(* Logix 5000 AddOnInstructionDefinition export MIS_COM; software revision 33.00 *)

TYPE JVL_AXIS_MIS :   // Drive Data
STRUCT
   ActualMode : DINT;
   ActualPosition : REAL;   // P_IST
   ActualVelocity : REAL;   // V_IST(16)
   ActualTorque : REAL;   // ACTUAL_TORQUE
   AxisStatus : JVL_MIS_STATUS;
   AxisWarnings : JVL_MIS_Warnings;
   AxisError : JVL_MIS_Error;
   RequestedMode : DINT;
   RequestedPosition : DINT;   // P_SOLL
   RequestedVelocity : DINT;   // V_SOLL
   RequestedAcceleration : DINT;   // A_SOLL
   RequestedDeceleration : DINT;
   GeneralCommand : DINT;
   CommandTorque : REAL;   // Requested Torque, T_SOLL
   ZeroSearchVelocity : REAL;   // Homing velocity
   ZeroSearchPosition : REAL;   // Homing position
   ZeroSearchTorque : DINT;   // Homing torque setpoint threshold value
   ZeroSearchTThreshold : DINT;   // Threshold for torque zerosearch trigger, usually 20% lower than running torque
   TravelConst : REAL;   // Factor to multiply P_IST and P_SOLL for scaling
   VelConst : REAL;   // Factor to multiply V_SOLL and V_IST to get scaled velocity value
   HomingType : DINT;   // Holds the reqested homingtype
   LoadFactor : DINT;   // Inertia ratio motor/load
   Configured : DINT;
   MSG_OutValue : DINT;   // Used in exp. output message to the motor
   MSG_InValue : DINT;   // Used in Exp. output message, to get value from motor
   MSG_OutInstance : DINT;   // Registernumber
   MSG_InInstance : DINT;   // Registernummer
   V_SOLL_CountsPerSample : REAL;
   AOI_Type : DINT;   // MIS_Disable = 1, MIS_Home = 2, MIS_Jog = 3, MIS_Position = 4, MIS_Reset = 5, MIS_Stop = 6
   Position_AppType : REAL;   // Position depending on the Application type
   MSG_Out_Execute : BOOL;   // Enable MSG_Out
   MSG_In_Execute : BOOL;   // Enable MSG_In
   ErrorReset : BOOL;
   MSG_Out_Busy : BOOL;
   MSG_In_Busy : BOOL;
   MSG_Out_Done : BOOL;
   MSG_In_Done : BOOL;
END_STRUCT
END_TYPE

TYPE JVL_MIS_Error :
STRUCT
   GeneralError : BOOL;
   FollowingError : BOOL;
   OutputDriver : BOOL;
   PositionLimit : BOOL;
   LowBusVoltage : BOOL;
   OverVoltage : BOOL;
   TemperatureLimit : BOOL;
   Internal : BOOL;
   AbsoluteMultiturnEncoderPositionLost : BOOL;
   AbsoluteMultiturnEncoderSensorCounting : BOOL;
   AbsoluteMultiturnEncoderCommsFailed : BOOL;
   SSIEncoderCounting : BOOL;
   ClosedLoop : BOOL;
   ExternalMemory : BOOL;
   AbsoluteSingleturnEncoder : BOOL;
   H4InternalEncoderError : BOOL;
   ZeroSearchTimeout : BOOL;
   CVIUnstable : BOOL;
   MotorDriverOverload : BOOL;
   Reserved_19 : BOOL;
   Reserved_20 : BOOL;
   Reserved_21 : BOOL;
   Reserved_22 : BOOL;
   Reserved_23 : BOOL;
   Reserved_24 : BOOL;
   Reserved_25 : BOOL;
   Reserved_26 : BOOL;
   STO_Alarm : BOOL;
   Reserved_28 : BOOL;
   STO : BOOL;
   Reserved_30 : BOOL;
   Reserved_31 : BOOL;
END_STRUCT
END_TYPE

TYPE JVL_MIS_STATUS :   // STATUS JVL Stepper
STRUCT
   Reserved_0 : BOOL;
   AutoCorrectionActive : BOOL;
   InPhysicalPosition : BOOL;
   AtVelocity : BOOL;
   InPosition : BOOL;
   Accelerating : BOOL;
   Decelerating : BOOL;
   ZeroSearchDone : BOOL;
   PasswordLock : BOOL;
   MagneticEncoderError : BOOL;
   H3CalibrationDataPresent : BOOL;
   H3LinearisationTableRecorded : BOOL;
   GeneralError : BOOL;
   H3CalibrationDataLocked : BOOL;
   ElectromechBrakeActive : BOOL;
   ClosedLoopLeadLagDetected : BOOL;
   ClosedLoopActivated : BOOL;
   InternalEncoderCalibrated : BOOL;
   StandbyCurrentIsUsed : BOOL;
   STOEnabled : BOOL;
   InternalEncoderOK : BOOL;
   EthernetSyncActivated : BOOL;
   InTargetPosition : BOOL;
   STOChannelAOK : BOOL;
   STOChannelBOK : BOOL;
   External_memory_sizeA : BOOL;
   External_memory_sizeB : BOOL;
   Reserved_27 : BOOL;
   Reserved_28 : BOOL;
   Reserved_29 : BOOL;
   Reserved_30 : BOOL;
   Reserved_31 : BOOL;
END_STRUCT
END_TYPE

TYPE JVL_MIS_Warnings :
STRUCT
   PositiveLimitActive : BOOL;
   NegativeLimitActive : BOOL;
   PositiveLimitHasBeenReached : BOOL;
   NegativeLimitHasBeenReached : BOOL;
   LowBusVoltage : BOOL;
   Reserved_5 : BOOL;
   TemperatureWarning : BOOL;
   SSIEncoder : BOOL;
   DriverOverload : BOOL;
   STOActive : BOOL;
   Reserved_10 : BOOL;
   Reserved_11 : BOOL;
   Reserved_12 : BOOL;
   Reserved_13 : BOOL;
   Reserved_14 : BOOL;
   Reserved_15 : BOOL;
   Reserved_16 : BOOL;
   Reserved_17 : BOOL;
   Reserved_18 : BOOL;
   Reserved_19 : BOOL;
   Reserved_20 : BOOL;
   Reserved_21 : BOOL;
   Reserved_22 : BOOL;
   Reserved_23 : BOOL;
   Reserved_24 : BOOL;
   Reserved_25 : BOOL;
   Reserved_26 : BOOL;
   Reserved_27 : BOOL;
   Reserved_28 : BOOL;
   Reserved_29 : BOOL;
   Reserved_30 : BOOL;
   Reserved_31 : BOOL;
END_STRUCT
END_TYPE

ADD_ON_INSTRUCTION MIS_COM   (* revision 1.0 *)
VAR_IN_OUT
   JVL_IN : AB:ETHERNET_MODULE_DINT_32Bytes:I:0; {required}
   JVL_OUT : AB:ETHERNET_MODULE_DINT_32Bytes:O:0; {required}
   MSG_IN : MESSAGE; {required}
   MSG_OUT : MESSAGE; {required}
   AXIS : JVL_AXIS_MIS; {required}
END_VAR
VAR_INPUT
   TravelPerRev : REAL := 1.0; {required}   // Travel per Revolution. Exc. actuator w. 60mm/rev, then value=60
   GearRatio : REAL := 1.0; {required}   // Gear ratio if a gearbox is mounted. select 1 for none
   ApplicationType : DINT; {required}   // Application_Type - 0=none (counts) 1=linear 2=degree
END_VAR
VAR
   CountsPerRevolution : REAL; {access None}
   vel : INT; {access None}
   torque : INT; {access None}
END_VAR

ROUTINE Logic   (* structured text *)
   
   
   	    AXIS.V_SOLL_CountsPerSample := 100.0;
   		CountsPerRevolution:= 409600.0;
   
   
   	//counts
   	if ApplicationType = 0 then
   	AXIS.TravelConst := 1;
   	AXIS.VelConst:= AXIS.V_SOLL_CountsPerSample;
   	//linear
   	elsif ApplicationType = 1 then
   	AXIS.TravelConst :=(CountsPerRevolution * GearRatio) / TravelPerRev;
   	AXIS.VelConst:= AXIS.V_SOLL_CountsPerSample * 60 * GearRatio / TravelPerRev;
   	//360°
   	elsif ApplicationType = 2 then
   	AXIS.TravelConst :=(CountsPerRevolution * GearRatio) / 360;
   	AXIS.VelConst:= AXIS.V_SOLL_CountsPerSample * 60 * GearRatio / 360;
   	end_if;
   
   
   AXIS.ActualMode := JVL_IN.Data[0];
   AXIS.ActualPosition := JVL_IN.Data[1];
   AXIS.ActualVelocity := JVL_IN.Data[2]/AXIS.VelConst;
   
   AXIS.ActualTorque := abs(JVL_IN.Data[6]) *0.049; //* 100 / 2047;
   
   AXIS.Position_AppType := AXIS.ActualPosition /AXIS.TravelConst;
   JVL_OUT.Data[0]:= AXIS.RequestedMode;
   //cop(AXIS.RequestedPosition,JVL_OUT.Data[1],4);
   JVL_OUT.Data[1]:= AXIS.RequestedPosition;
   //cop(AXIS.RequestedVelocity,JVL_OUT.Data[2],4);
   JVL_OUT.Data[2]:= AXIS.RequestedVelocity;
   JVL_OUT.Data[3]:= AXIS.RequestedAcceleration;
   JVL_OUT.Data[4]:= AXIS.RequestedDeceleration;
   JVL_OUT.Data[5]:= AXIS.GeneralCommand;
   
   AXIS.MSG_Out_Done:= MSG_OUT.DN;
   AXIS.MSG_Out_Busy:= MSG_OUT.EN;
   AXIS.MSG_In_Done:= MSG_IN.DN;
   AXIS.MSG_In_Busy:= MSG_IN.EN;
   
   MSG_OUT.Instance:= AXIS.MSG_OutInstance;
   MSG_IN.Instance:= AXIS.MSG_InInstance;
   //Status
     AXIS.AxisStatus.STOChannelBOK := JVL_IN.Data[3].24;
     AXIS.AxisStatus.External_memory_sizeA := JVL_IN.Data[3].25;
     AXIS.AxisStatus.External_memory_sizeB := JVL_IN.Data[3].26;
     AXIS.AxisStatus.Reserved_27 := JVL_IN.Data[3].27;
     AXIS.AxisStatus.Reserved_28 := JVL_IN.Data[3].28;
     AXIS.AxisStatus.Reserved_29 := JVL_IN.Data[3].29;
     AXIS.AxisStatus.Reserved_30 := JVL_IN.Data[3].30;
     AXIS.AxisStatus.Reserved_31 := JVL_IN.Data[3].31;
     AXIS.AxisStatus.ClosedLoopActivated := JVL_IN.Data[3].16;
     AXIS.AxisStatus.InternalEncoderCalibrated := JVL_IN.Data[3].17;
     AXIS.AxisStatus.StandbyCurrentIsUsed := JVL_IN.Data[3].18;
     AXIS.AxisStatus.STOEnabled := JVL_IN.Data[3].19;
     AXIS.AxisStatus.InternalEncoderOK := JVL_IN.Data[3].20;
     AXIS.AxisStatus.EthernetSyncActivated := JVL_IN.Data[3].21;
     AXIS.AxisStatus.InTargetPosition := JVL_IN.Data[3].22;
     AXIS.AxisStatus.STOChannelAOK := JVL_IN.Data[3].23;
     AXIS.AxisStatus.PasswordLock := JVL_IN.Data[3].8;
     AXIS.AxisStatus.MagneticEncoderError := JVL_IN.Data[3].9;
     AXIS.AxisStatus.H3CalibrationDataPresent := JVL_IN.Data[3].10;
     AXIS.AxisStatus.H3LinearisationTableRecorded := JVL_IN.Data[3].11;
     AXIS.AxisStatus.GeneralError := JVL_IN.Data[3].12;
     AXIS.AxisStatus.H3CalibrationDataLocked := JVL_IN.Data[3].13;
     AXIS.AxisStatus.ElectromechBrakeActive := JVL_IN.Data[3].14;
     AXIS.AxisStatus.ClosedLoopLeadLagDetected := JVL_IN.Data[3].15;
     AXIS.AxisStatus.Reserved_0 := JVL_IN.Data[3].0;
     AXIS.AxisStatus.AutoCorrectionActive := JVL_IN.Data[3].1;
     AXIS.AxisStatus.InPhysicalPosition := JVL_IN.Data[3].2;
     AXIS.AxisStatus.AtVelocity := JVL_IN.Data[3].3;
     AXIS.AxisStatus.InPosition := JVL_IN.Data[3].4;
     AXIS.AxisStatus.Accelerating := JVL_IN.Data[3].5;
     AXIS.AxisStatus.Decelerating := JVL_IN.Data[3].6;
     AXIS.AxisStatus.ZeroSearchDone := JVL_IN.Data[3].7;
   
     //Warnings
   AXIS.AxisWarnings.PositiveLimitActive := JVL_IN.Data[4].0;
   AXIS.AxisWarnings.NegativeLimitActive := JVL_IN.Data[4].1;
   AXIS.AxisWarnings.PositiveLimitHasBeenReached := JVL_IN.Data[4].2;
   AXIS.AxisWarnings.NegativeLimitHasBeenReached := JVL_IN.Data[4].3;
   AXIS.AxisWarnings.LowBusVoltage := JVL_IN.Data[4].4;
   AXIS.AxisWarnings.Reserved_5 := JVL_IN.Data[4].5;
   AXIS.AxisWarnings.TemperatureWarning := JVL_IN.Data[4].6;
   AXIS.AxisWarnings.SSIEncoder := JVL_IN.Data[4].7;
   AXIS.AxisWarnings.DriverOverload := JVL_IN.Data[4].8;
   AXIS.AxisWarnings.STOActive := JVL_IN.Data[4].9;
   
   //ErrorsAXIS.AxisError.Reserved_24 := JVL_IN.Data[5].24;
   AXIS.AxisError.Reserved_25 := JVL_IN.Data[5].25;
   AXIS.AxisError.Reserved_26 := JVL_IN.Data[5].26;
   AXIS.AxisError.STO_Alarm := JVL_IN.Data[5].27;
   AXIS.AxisError.Reserved_28 := JVL_IN.Data[5].28;
   AXIS.AxisError.STO := JVL_IN.Data[5].29;
   AXIS.AxisError.Reserved_30 := JVL_IN.Data[5].30;
   AXIS.AxisError.Reserved_31 := JVL_IN.Data[5].31;
   AXIS.AxisError.ZeroSearchTimeout := JVL_IN.Data[5].16;
   AXIS.AxisError.CVIUnstable := JVL_IN.Data[5].17;
   AXIS.AxisError.MotorDriverOverload := JVL_IN.Data[5].18;
   AXIS.AxisError.Reserved_19 := JVL_IN.Data[5].19;
   AXIS.AxisError.Reserved_20 := JVL_IN.Data[5].20;
   AXIS.AxisError.Reserved_21 := JVL_IN.Data[5].21;
   AXIS.AxisError.Reserved_22 := JVL_IN.Data[5].22;
   AXIS.AxisError.Reserved_23 := JVL_IN.Data[5].23;
   AXIS.AxisError.AbsoluteMultiturnEncoderPositionLost := JVL_IN.Data[5].8;
   AXIS.AxisError.AbsoluteMultiturnEncoderSensorCounting := JVL_IN.Data[5].9;
   AXIS.AxisError.AbsoluteMultiturnEncoderCommsFailed := JVL_IN.Data[5].10;
   AXIS.AxisError.SSIEncoderCounting := JVL_IN.Data[5].11;
   AXIS.AxisError.ClosedLoop := JVL_IN.Data[5].12;
   AXIS.AxisError.ExternalMemory := JVL_IN.Data[5].13;
   AXIS.AxisError.AbsoluteSingleturnEncoder := JVL_IN.Data[5].14;
   AXIS.AxisError.H4InternalEncoderError := JVL_IN.Data[5].15;
   AXIS.AxisError.GeneralError := JVL_IN.Data[5].0;
   AXIS.AxisError.FollowingError := JVL_IN.Data[5].1;
   AXIS.AxisError.OutputDriver := JVL_IN.Data[5].2;
   AXIS.AxisError.PositionLimit := JVL_IN.Data[5].3;
   AXIS.AxisError.LowBusVoltage := JVL_IN.Data[5].4;
   AXIS.AxisError.OverVoltage := JVL_IN.Data[5].5;
   AXIS.AxisError.TemperatureLimit := JVL_IN.Data[5].6;
   AXIS.AxisError.Internal := JVL_IN.Data[5].7;
   
END_ROUTINE
END_ADD_ON_INSTRUCTION

ADD_ON_INSTRUCTION MIS_Disable   (* revision 1.0 *)
VAR_IN_OUT
   AXIS : JVL_AXIS_MIS; {required}
END_VAR
VAR_OUTPUT
   Busy : BOOL; {access Read Only, visible}
   CommandAborted : BOOL; {access Read Only, visible}
   Done : BOOL; {access Read Only, visible}
   Error : BOOL; {access Read Only, visible}
END_VAR
VAR_INPUT
   Execute : BOOL; {required}
END_VAR
VAR
   State : INT; {access None}
   ExecuteStart : BOOL; {access None}
   AOI_Type : DINT; {access None}
END_VAR

ROUTINE Logic   (* structured text *)
   	//REGION CAPTURE EDGES
   	    if Execute and not ExecuteStart then
   	    	ExecuteStart:=1;
   		elsif not Execute then
   			ExecuteStart:=0;
   		end_if;
   
   	//END_REGION
   
   	//REGION STATE CHANGES
   
   	    //Re-trigger sequence from start on rising edge
   
   	    //Command aborted
   	    IF AXIS.AOI_Type <> AOI_Type AND
   	        State <> 0 AND
   	        State <> 90 AND
   	        State <> 30 AND
   	        State <> 80
   	    THEN
   	        State := 80;
   	    END_IF;
   
   
   	    //Error if motor error while executing
   	    IF AXIS.AxisError.GeneralError AND
   	        State <> 0 AND
   	        State <> 90 AND
   	        State <> 20 AND
   	        State <> 80
   	    THEN
   	        State := 90;
   	    END_IF;
   
   	//END_REGION
   
   	//REGION STATE MACHINE
   
   	    CASE State OF
   
   	        0:        //Wait for rising edge on execute
   	            IF ExecuteStart THEN
   					AOI_Type:= 1;
   					AXIS.AOI_Type:= 1;
   	                State := 10;
   	            END_IF;
   
   	        10:     //Put JVL into passive state
   	            AXIS.RequestedMode:= 0;
   	            IF AXIS.ActualMode = 0 THEN
   	                State := 20;
   	            END_IF;
   
   	        20:        //Disable complete, reset to idle by setting execute false
   	            IF NOT Execute THEN
   	                State := 0;
   	            END_IF;
   
   	        80:     //Aborted by other command before completion
   	            IF NOT Execute THEN
   	                State := 0;
   	            END_IF;
   
   	        90:       //Error while disabling, reset to idle by setting execute false
   	            IF NOT Execute THEN
   	                State := 0;
   	            END_IF;
   
   	        ELSE
   	            State := 90;
   
   	    END_CASE;
   
   	//END_REGION
   
   	//REGION STATUS SIGNALS
   
   	    Done := State = 20;
   	    CommandAborted := State = 80;
   	    Error := State = 90;
   	    Busy := State <> 0 AND NOT Done AND NOT Error AND NOT CommandAborted;
   
   	//END_REGION
   
END_ROUTINE
END_ADD_ON_INSTRUCTION

ADD_ON_INSTRUCTION MIS_Home   (* revision 1.0 *)
VAR_IN_OUT
   Axis : JVL_AXIS_MIS; {required}
END_VAR
VAR_OUTPUT
   Busy : BOOL; {access Read Only, visible}
   CommandAborted : BOOL; {access Read Only, visible}
   Done : BOOL; {access Read Only, visible}
   Error : BOOL; {access Read Only, visible}
END_VAR
VAR_INPUT
   Execute : BOOL; {required}
   Mode : INT; {required}
   Position : REAL; {required}
   Offset : REAL; {required}
   Velocity : REAL; {required}
   VelocityReduced : REAL; {required}
   Acceleration : REAL; {required}
   Deceleration : REAL; {required}
   TorqueLimit : REAL; {required}
END_VAR
VAR
   State : INT; {access None}
   ActiveMode : INT; {access None}
   Mode0State : INT; {access None}
   Mode1State : INT; {access None}
   ActivePosition : REAL; {access None}
   ActiveVelocity : REAL; {access None}
   ActiveAcceleration : REAL; {access None}
   ActiveTorqueLimit : REAL; {access None}
   ActiveOffset : REAL; {access None}
   Mode2State : INT; {access None}
   Mode3State : INT; {access None}
   ExecuteStart : BOOL; {access None}
   Ton_wait : FBD_TIMER; {access None}
   AOI_Type : DINT; {access None}
   ActiveVelocityReduced : REAL;
   ActiveDeceleration : DINT; {access None}
END_VAR

ROUTINE Logic   (* structured text *)
   	//REGION CAPTURE EDGES
   	    if Execute and not ExecuteStart then
   	    	ExecuteStart:=1;
   		elsif not Execute then
   			ExecuteStart:=0;
   		end_if;
   
   	//END_REGION
   
   	//REGION STATE CHANGES
   
   	    //Re-trigger sequence from start on rising edge
   
   
   	    //Command aborted
   	    IF Axis.AOI_Type <> AOI_Type AND
   	        State <> 0 AND
   	        State <> 90 AND
   	        State <> 30 AND
   	        State <> 80
   	    THEN
   	        State := 80;
   	    END_IF;
   
   
   	    //Error if motor error while executing
   	    IF Axis.AxisError.GeneralError AND
   	        State <> 0 AND
   	        State <> 90 AND
   	        State <> 30 AND
   	        State <> 80
   	    THEN
   	        State := 90;
   	    END_IF;
   	//END_REGION
   
   	//REGION STATE MACHINE
   
   
   
   	    CASE State OF
   
   	        0:
   	            //Reset static values
   	            ActiveMode := 0;
   	            ActivePosition := 0;
   	            ActiveVelocity := 0;
   	            ActiveVelocityReduced:=0;
   				ActiveAcceleration := 0;
   	            ActiveDeceleration := 0;
   				ActiveTorqueLimit := 0;
   	            ActiveOffset := 0;
   
   	            //Reset mode states
   	            Mode0State := 0;
   	            Mode1State := 0;
   	            Mode2State := 0;
   	            Mode3State := 0;
   
   	            IF ExecuteStart THEN
   					//
   					AOI_Type:= 2;
   					Axis.AOI_Type:= 2;
   	                //
   					Axis.GeneralCommand := 0;
   	                ActiveMode := Mode;
   	                ActivePosition := Position * Axis.TravelConst;
   	                ActiveVelocity := Velocity * Axis.VelConst;// * Axis.Device.Config.V_SOLL_CountsPerSample);
   	                ActiveVelocityReduced := VelocityReduced * Axis.VelConst;// * Axis.Device.Config.V_SOLL_CountsPerSample);
   	                ActiveAcceleration := ABS(Acceleration) ;
   	                ActiveDeceleration := ABS(Deceleration) ;
   	                //set Acceleration always >=1
   	                IF ActiveAcceleration < 1 THEN
   	                    ActiveAcceleration := 1;
   	                END_IF;
   
   	                ActiveTorqueLimit := TorqueLimit * 2047/100;
   	                ActiveOffset := Offset * Axis.TravelConst;
   
   	                State := 10;
   	            END_IF;
   
   	        10:
   	            // change to velocity mode with zero setpoint to ensure motor does not run off to current position when homed
   	            IF ActiveAcceleration < 1 THEN
   	                Axis.RequestedAcceleration := 1;
   	            ELSE
   	                Axis.RequestedAcceleration := ActiveAcceleration;
   	                Axis.RequestedDeceleration := ActiveDeceleration;
   
   	            END_IF;
   	            Axis.RequestedVelocity := 0;
   	            Axis.RequestedMode := 1;
   	            // change position setpoint to new home position
   	            Axis.RequestedPosition := ActivePosition;
   	            // reset register trigger
   	            Axis.MSG_Out_Execute := 0;
   	            Axis.MSG_In_Execute := 0;
   	            // start homing
   	            State := 20;
   
   	        20:
   	            CASE ActiveMode OF
   
   	                0:  // Set Home Position
   	                    CASE Mode0State OF
   	                        0:
   
   								Axis.MSG_OutInstance := 144;
   
   	                            Axis.MSG_OutValue:=Position;
   	                            Axis.MSG_Out_Execute := 1;
   	                            Axis.GeneralCommand := 16#0;
   	                            IF Axis.MSG_Out_Busy AND NOT Axis.MSG_Out_Done THEN
   	                                Mode0State := 10;
   	                            END_IF;
   	                        10:
   	                            IF Axis.MSG_Out_Done THEN
   	                                Axis.MSG_Out_Execute := 0;
   	                                Mode0State := 20;
   	                            END_IF;
   	                        20:
   	                            Axis.GeneralCommand := 16#80000162;//16#1000162 also
   	                            IF ABS(Axis.ActualPosition - Position) < 50.0 THEN
   	                                Mode0State := 30;
   	                            END_IF;
   	                        30:
   	                            Axis.GeneralCommand := 16#0;
   	                            Mode0State := 50;
   	                        50:
   	                            State := 30;
   	                        ELSE
   	                            State := 90;
   	                    END_CASE;
   
   	                1:  // Home to Sensor (type 2, bidirectional)
   	                    CASE Mode1State OF
   	                       0:
   	                            // set home position offset move distance
   
   		                            Axis.MSG_OutInstance := 38;
   		                            Axis.MSG_OutValue := ActiveOffset;
   		                            Axis.MSG_Out_Execute := 1;
   		                            IF Axis.MSG_Out_Busy THEN
   		                                Mode1State := 5;
   		                            END_IF;
   
   	                        5:
   
   	                            IF Axis.MSG_Out_Done THEN
   	                                Axis.MSG_Out_Execute := 0;
   	                                Mode1State := 10;
   	                            END_IF;
   	                       10:
   	                            //homing velocity
   	                            Axis.MSG_OutInstance := 40;
   	                            Axis.MSG_OutValue:=ActiveVelocity;
   
   	                            Axis.MSG_Out_Execute := 1;
   	                            IF Axis.MSG_Out_Busy THEN
   	                                Mode1State := 15;
   	                            END_IF;
   	                       15:
   	                            IF Axis.MSG_Out_Done THEN
   	                                Axis.MSG_Out_Execute := 0;
   	                                Mode1State := 20;
   	                            END_IF;
   
   	                       20:
   	                            // set homing reduced/crawl velocity
   	                            Axis.MSG_OutInstance := 242;
   	                            Axis.MSG_OutValue:=ActiveVelocityReduced;
   	                            Axis.MSG_Out_Execute := 1;
   	                            IF Axis.MSG_Out_Busy THEN
   	                                Mode1State := 30;
   	                            END_IF;
   	                        30:
   	                            IF Axis.MSG_Out_Done THEN
   	                                Axis.MSG_Out_Execute := 0;
   	                                Mode1State := 60;
   	                            END_IF;
   	                        60:
   	                            // start homing mode
   	                            Axis.RequestedMode := 14;
   
   	                            // homing done
   	                            IF NOT Axis.AxisStatus.ZeroSearchDone THEN
   	                                Mode1State := 70;
   	                            END_IF;
   	                        70:
   	                            IF Axis.AxisStatus.ZeroSearchDone THEN
   	                                Axis.RequestedVelocity := 0;
   	                                Axis.RequestedMode := 2;
   	                                Mode1State := 80;
   	                            END_IF;
   	                        80:
   	                            State := 30;
   	                        ELSE
   	                            State := 90;
   	                    END_CASE;
   
   	                2:  // Home to Endstop (torque limit)
   	                    CASE Mode2State OF
   	                        0:
   	                            //Home to Endstop (torque limit);
   								Axis.MSG_OutInstance := 38;
   	                            Axis.MSG_OutValue := ActiveOffset;
   	                            Axis.MSG_Out_Execute := 1;
   
   	                            IF Axis.MSG_Out_Busy THEN
   	                                Mode2State := 15;
   	                            END_IF;
   	                        15:
   	                            IF Axis.MSG_Out_Done THEN
   	                                Axis.MSG_Out_Execute := 0;
   	                                Mode2State := 20;
   	                            END_IF;
   	                        20:
   								Axis.MSG_OutInstance := 40;
   	                            Axis.MSG_OutValue := ActiveVelocity;// * Axis.Device.Config.V_SOLL_CountsPerSample;
   	                            Axis.MSG_Out_Execute := 1;
   	                            IF Axis.MSG_Out_Busy THEN
   	                                Mode2State := 25;
   	                            END_IF;
   	                        25:
   	                            IF Axis.MSG_Out_Done THEN
   	                                Axis.MSG_Out_Execute := 0;
   	                                Mode2State := 34;
   
   	                            END_IF;
   	                        34:
   								Axis.MSG_OutInstance := 41;
   	                            Axis.MSG_OutValue := ActiveTorqueLimit;
   	                            Axis.MSG_Out_Execute := 1;
   
   	                            IF Axis.MSG_Out_Busy THEN
   	                                Mode2State := 37;
   	                            END_IF;
   	                        37:
   	                            IF Axis.MSG_Out_Done THEN
   	                                Axis.MSG_Out_Execute := 0;
   	                                Mode2State := 40;
   	                            END_IF;
   	                        40:
   	                            Axis.RequestedMode := 12;
   	                            // homing done-register 42 Homemode bit 16
   	                            IF NOT Axis.AxisStatus.ZeroSearchDone THEN
   	                                Mode2State := 45;
   	                            END_IF;
   	                        45:
   	                            IF Axis.AxisStatus.ZeroSearchDone THEN
   	                                Axis.RequestedVelocity := 0;
   	                                Axis.RequestedMode := 2;
   	                                Mode2State := 60;
   	                            END_IF;
   
   	                        60:
   	                            State := 30;
   	                        ELSE
   	                            State := 90;
   	                    END_CASE;
   
   
   
   	            END_CASE;
   
   	        30:        //Home complete, reset to idle by setting execute false
   	            IF NOT Execute THEN
   	                State := 0;
   	            END_IF;
   
   	        80:     //Aborted by other command before completion
   	            IF NOT Execute THEN
   	                State := 0;
   	            END_IF;
   
   	        90:       //Error while disabling, reset to idle by setting execute false
   	            IF NOT Execute THEN
   	                State := 0;
   	            END_IF;
   
   	        ELSE
   	            State := 90;
   
   	    END_CASE;
   
   	//END_REGION
   
   	//REGION STATUS SIGNALS
   
   	    Done := State = 30;
   	    CommandAborted := State = 80;
   	    Error := State = 90;
   	    Busy := State <> 0 AND NOT Done AND NOT Error AND NOT CommandAborted;
   
   	//END_REGION
END_ROUTINE
END_ADD_ON_INSTRUCTION

ADD_ON_INSTRUCTION MIS_Jog   (* revision 1.0 *)
VAR_IN_OUT
   AXIS : JVL_AXIS_MIS; {required}
END_VAR
VAR_INPUT
   JogForwards : BOOL; {required}
   JogBackwards : BOOL; {required}
END_VAR
VAR_OUTPUT
   Busy : BOOL; {access Read Only, visible}
   CommandAborted : BOOL; {access Read Only, visible}
   AtVelocity : BOOL; {access Read Only, visible}
   Error : BOOL; {access Read Only, visible}
END_VAR
VAR_INPUT
   Acceleration : REAL; {required}
   Deceleration : REAL; {required}
   Velocity : REAL; {required}
END_VAR
VAR
   ForwardStart : BOOL; {access None}
   BackwardStart : BOOL; {access None}
   State : INT; {access None}
   ActiveVelocity : REAL; {access None}
   ActiveAcceleration : REAL; {access None}
   AOI_Type : DINT; {access None}
   ActiveDeceleration : DINT; {access None}
END_VAR

ROUTINE Logic   (* structured text *)
   	//REGION CAPTURE EDGES
   	    if JogForwards and not ForwardStart then
   	    	ForwardStart:=1;
   	    elsif JogBackwards  and not BackwardStart then
   	    	BackwardStart:=1;
   		elsif not JogForwards and not JogBackwards then
   			ForwardStart:=0;
   	    	BackwardStart:=0;
   		end_if;
   
   	//END_REGION
   
   	//REGION STATE CHANGES
   
   	    //Re-trigger sequence from start on rising edge
   	    //Command aborted
   	    IF AXIS.AOI_Type <> AOI_Type AND
   	        State <> 0 AND
   	        State <> 90 AND
   	        State <> 80
   	    THEN
   	        State := 80;
   	    END_IF;
   
   
   
   	    //Error if motor error while executing
   	    IF AXIS.AxisError.GeneralError AND
   	        State <> 0 AND
   	        State <> 90 AND
   	        State <> 80
   	    THEN
   	        State := 90;
   	    END_IF;
   
   	//END_REGION
   
   	//REGION STATE MACHINE
   
   	    CASE State OF
   
   	        0:
   	            ActiveVelocity := 0;
   	            ActiveAcceleration := 0;
   	            ActiveDeceleration := 0 ;
   
   	            IF ForwardStart OR BackwardStart THEN
   					AOI_Type:= 3;
   					AXIS.AOI_Type:= 3;
   	                AXIS.RequestedMode:= 1;
   	                ActiveAcceleration := ABS(Acceleration);
   	                ActiveDeceleration := ABS(Deceleration) ;
   	                //set Acceleration always >=1
   	                IF ActiveAcceleration < 1 THEN
   	                    ActiveAcceleration := 1;
   	                END_IF;
   	                IF JogForwards AND not JogBackwards THEN
   	                    ActiveVelocity := ABS(Velocity) * AXIS.VelConst;// * Axis.Device.Config.V_SOLL_CountsPerSample));
   	                    State := 10;
   	                ELSIF JogBackwards AND NOT JogForwards THEN
   	                    ActiveVelocity := -1.0 * ABS(Velocity)* AXIS.VelConst;// * Axis.Device.Config.V_SOLL_CountsPerSample));
   	                    State := 10;
   	                ELSE
   	                    State := 30;
   	                END_IF;
   
   	                State := 10;
   	            END_IF;
   
   	        10:
   	            IF AXIS.ActualMode = 1 THEN
   
   	                AXIS.RequestedAcceleration := ActiveAcceleration;
   	                AXIS.RequestedDeceleration := ActiveDeceleration;
   	                AXIS.RequestedVelocity := ActiveVelocity;
   
   	                IF JogForwards AND NOT JogBackwards THEN
   	                    State := 20;
   	                ELSIF JogBackwards AND NOT JogForwards THEN
   	                    State := 25;
   	                ELSE
   	                    State := 30;
   	                END_IF;
   
   	            END_IF;
   
   	        20:
   	            IF AXIS.ActualMode = 1 THEN
   
   	                IF NOT (JogForwards and not JogBackwards) THEN
   	                    State := 30;
   	                END_IF;
   
   	            ELSE
   	                State := 80;
   	            END_IF;
   
   	        25:
   	            IF AXIS.ActualMode = 1 THEN
   
   	                IF NOT (JogBackwards AND NOT JogForwards) THEN
   	                    State := 30;
   	                END_IF;
   
   	            ELSE
   	                State := 80;
   	            END_IF;
   
   	        30:
   	            AXIS.RequestedMode := 1;
   	            AXIS.RequestedVelocity := 0;
   
   	            State := 40;
   
   	        40:
   	            IF AXIS.ActualMode = 1  THEN
   
   	                //If no motion then stop is complete
   	                IF ABS((AXIS.ActualVelocity)) <= 1.0 AND
   	                    //not AXIS.AxisStatus.AtVelocity AND
   	                    NOT AXIS.AxisStatus.Accelerating AND
   	                    NOT AXIS.AxisStatus.Decelerating THEN
   	                    State := 0;
   	                END_IF;
   
   	            ELSE
   	                State := 80;
   	            END_IF;
   
   	        80:     //Aborted by other command before completion
   	            IF NOT JogForwards AND NOT JogBackwards THEN
   	                State := 0;
   	            END_IF;
   
   	        90:       //Error while jogging, reset to idle by setting jog inputs false
   	            IF NOT JogForwards AND NOT JogBackwards THEN
   	                State := 0;
   	            END_IF;
   
   	        ELSE
   	            State := 90;
   
   	    END_CASE;
   
   	//END_REGION
   
   	//REGION STATUS SIGNALS
   
   	    AtVelocity:=(State=20 or State = 25) AND
   	                      //AXIS.AxisStatus.AtVelocity AND
   	                      NOT AXIS.AxisStatus.Accelerating AND
   	                      NOT AXIS.AxisStatus.Decelerating;
   	    CommandAborted := State = 80;
   	    Error := State = 90;
   	    Busy := State <> 0 AND NOT Error AND NOT CommandAborted;
   
   	//END_REGION
   
END_ROUTINE
END_ADD_ON_INSTRUCTION

ADD_ON_INSTRUCTION MIS_Position   (* revision 1.0 *)
VAR_IN_OUT
   Axis : JVL_AXIS_MIS; {required}
END_VAR
VAR_OUTPUT
   Busy : BOOL; {access Read Only, visible}
   CommandAborted : BOOL; {access Read Only, visible}
   Done : BOOL; {access Read Only, visible}
   Error : BOOL; {access Read Only, visible}
END_VAR
VAR_INPUT
   Execute : BOOL; {required}
   Position : REAL; {required}
   Velocity : REAL; {required}
   Acceleration : REAL; {required}
   Deceleration : REAL; {required}
   AbsolutePositioning : BOOL; {required}
END_VAR
VAR
   State : INT; {access None}
   ExecuteStart : BOOL; {access None}
   ActiveAbsolute : BOOL; {access None}
   ActiveVelocity : REAL; {access None}
   ActiveAcceleration : REAL; {access None}
   ActiveTargetPosition : REAL; {access None}
   StartPosition : REAL; {access None}
   AOI_Type : DINT; {access None}
   ActiveDeceleration : DINT; {access None}
END_VAR

ROUTINE Logic   (* structured text *)
   	//REGION CAPTURE EDGES
   	    if Execute and not ExecuteStart then
   	    	ExecuteStart:=1;
   		elsif not Execute then
   			ExecuteStart:=0;
   		end_if;
   
   	//END_REGION
   
   	//REGION STATE CHANGES
   
   	    //Re-trigger sequence from start on rising edge
   
   
   	    //Command aborted
   	    IF Axis.AOI_Type <> AOI_Type AND
   	        State <> 0 AND
   	        State <> 90 AND
   	        State <> 30 AND
   	        State <> 80
   	    THEN
   	        State := 80;
   	    END_IF;
   
   
   	    //Error if motor error while executing
   	    IF Axis.AxisStatus.GeneralError AND
   	        State <> 0 AND
   	        State <> 90 AND
   	        State <> 30 AND
   	        State <> 80
   	    THEN
   	        State := 90;
   	    END_IF;
   	//END_REGION
   
   	//REGION STATE MACHINE
   
   	    CASE State OF
   
   	        0:
   	            ActiveVelocity := 0;
   	            ActiveAcceleration := 0;
   	            ActiveDeceleration := 0;
   				ActiveAbsolute := 0;
   	            ActiveTargetPosition := 0;
   
   	            IF ExecuteStart THEN
   					AOI_Type:= 4;
   					Axis.AOI_Type:= 4;
   	                Axis.RequestedMode := 2;
   	                StartPosition := Axis.ActualPosition;
   	                ActiveVelocity := ABS(Velocity) * Axis.VelConst;// * Axis.Device.Config.V_SOLL_CountsPerSample);
   	                ActiveAcceleration := ABS(Acceleration);
   	                ActiveDeceleration := ABS(Deceleration) ;
   	                //set Acceleration always >=1
   	                IF ActiveAcceleration < 1.0 THEN
   	                    ActiveAcceleration := 1.0;
   	                END_IF;
   
   	                ActiveAbsolute := AbsolutePositioning;
   
   	                IF ActiveAbsolute THEN
   	                    ActiveTargetPosition := Position *Axis.TravelConst;
   	                ELSE
   	                    ActiveTargetPosition := Position *Axis.TravelConst+ StartPosition;
   	                END_IF;
   
   	                State := 10;
   	            END_IF;
   
   	        10:
   	            IF Axis.ActualMode = 2 THEN
   	                Axis.RequestedAcceleration := ActiveAcceleration;
   	                Axis.RequestedDeceleration := ActiveDeceleration;
   	                Axis.RequestedPosition := ActiveTargetPosition;
   	                Axis.RequestedVelocity := ActiveVelocity;
   
   					State := 20;
   					(*
   	                IF ContinuousUpdate THEN
   	                    State := 25;
   	                ELSE
   	                    State := 20;
   	                END_IF;
   	                *)
   	            END_IF;
   
   	        20:
   	            IF Axis.ActualMode = 2 AND
   	                Axis.RequestedPosition = ActiveTargetPosition AND
   	                Axis.RequestedVelocity = ActiveVelocity THEN
   
   	                //If taget reached then move is complete
   	                IF ABS(ActiveTargetPosition - Axis.ActualPosition) <= 2000 AND
   	                    Axis.AxisStatus.InPosition AND
   	                    NOT Axis.AxisStatus.Accelerating AND
   	                    NOT Axis.AxisStatus.Decelerating THEN
   	                    State := 30;
   	                END_IF;
   
   	            ELSE
   	                State := 80;
   	            END_IF;
   
   	        30:
   	            IF NOT Execute THEN
   	                State := 0;
   	            END_IF;
   	        (*
   	        25:
   	            IF Axis.Telegram.Input.OperatingMode = 2 AND
   	                Axis.Telegram.Output.VelocitySetpoint = DINT_TO_DWORD(ActiveVelocity) AND
   	                Axis.Telegram.Output.PositionSetpoint = DINT_TO_DWORD(ActiveTargetPosition) THEN
   
   	                IF Execute THEN
   
   	                    ActiveVelocity := LREAL_TO_DINT(ABS(Velocity) * Axis.Device.Config.V_SOLL_CountsPerSample);
   	                    ActiveAcceleration := LREAL_TO_DINT(ABS(Acceleration) * Axis.Device.Config.A_SOLL_CountsPerSample2);
   	                    //set Acceleration always >=1
   	                    IF ActiveAcceleration < 1 THEN
   	                        ActiveAcceleration := 1;
   	                    END_IF;
   	                    IF ActiveAbsolute THEN
   	                        ActiveTargetPosition := Position;
   	                    ELSE
   	                        ActiveTargetPosition := Position + StartPosition;
   	                    END_IF;
   
   	                    Axis.Telegram.Output.AccelerationSetpoint := ActiveAcceleration;
   	                    Axis.Telegram.Output.PositionSetpoint := ActiveTargetPosition;
   	                    Axis.Telegram.Output.VelocitySetpoint := ActiveVelocity;
   
   	                    //If taget reached then move is complete
   	                    IF ABS(DINT_TO_LREAL(ActiveTargetPosition - Axis.Telegram.Input.ActualPosition)) <= 5.0 AND
   	                        Axis.Telegram.Input.StatusError.InPosition AND
   	                        NOT Axis.Telegram.Input.StatusError.Accelerating AND
   	                        NOT Axis.Telegram.Input.StatusError.Decelerating THEN
   	                        State := 35;
   	                    END_IF;
   
   	                ELSE
   	                    State := 20;
   	                END_IF;
   
   	            ELSE
   	                State := 80;
   	            END_IF;
   
   	        35:
   	            IF Execute THEN
   
   	                IF ActiveAbsolute THEN
   	                    IF ActiveTargetPosition <> Position THEN
   	                        State := 20;
   	                    END_IF;
   	                ELSE
   	                    IF ActiveTargetPosition <> (Position + StartPosition) THEN
   	                        State := 25;
   	                    END_IF;
   	                END_IF;
   
   	            ELSE
   	                State := 0;
   	            END_IF;
   	        *)
   	        80:     //Aborted by other command before completion
   	            IF NOT Execute THEN
   	                State := 0;
   	            END_IF;
   
   	        90:       //Error, reset to idle by setting execute false
   	            IF NOT Execute THEN
   	                State := 0;
   	            END_IF;
   	            //Mode=Passiv
   	            Axis.RequestedMode := 0;
   	        ELSE
   	            State := 90;
   
   	    END_CASE;
   
   	//END_REGION
   
   	//REGION STATUS SIGNALS
   
   	    Done := State = 30 OR State = 35;
   	    CommandAborted := State = 80;
   	    Error := State = 90;
   	    Busy := State <> 0 AND NOT Done AND NOT Error AND NOT CommandAborted;
   
   	//END_REGION
END_ROUTINE
END_ADD_ON_INSTRUCTION

ADD_ON_INSTRUCTION MIS_Reset   (* revision 1.0 *)
VAR_IN_OUT
   AXIS : JVL_AXIS_MIS; {required}
END_VAR
VAR_OUTPUT
   Busy : BOOL; {access Read Only, visible}
   CommandAborted : BOOL; {access Read Only, visible}
   Done : BOOL; {access Read Only, visible}
END_VAR
VAR_INPUT
   Execute : BOOL; {required}
END_VAR
VAR
   State : INT; {access None}
   ExecuteStart : BOOL; {access None}
   AOI_Type : DINT; {access None}
END_VAR

ROUTINE Logic   (* structured text *)
   	//REGION CAPTURE EDGES
   	    if Execute and not ExecuteStart then
   	    	ExecuteStart:=1;
   		elsif not Execute then
   			ExecuteStart:=0;
   		end_if;
   
   	//END_REGION
   
   	//REGION STATE CHANGES
   
   	    //Re-trigger sequence from start on rising edge
   	    //Command aborted
   	    IF AXIS.AOI_Type <> AOI_Type AND
   	        State <> 0 AND
   	        State <> 90 AND
   	        State <> 30 AND
   	        State <> 80
   	    THEN
   	        State := 80;
   	    END_IF;
   
   
   	//END_REGION
   
   	//REGION STATE MACHINE
   
   	    CASE State OF
   
   	        0:
   	            IF ExecuteStart THEN
   					AOI_Type:= 5;
   					AXIS.AOI_Type:= 5;
   	                AXIS.GeneralCommand := 16#0;
   	                State := 10;
   	            END_IF;
   
   	        10:
   	            AXIS.RequestedMode := 0;
   	            AXIS.RequestedAcceleration := 0;
   	            AXIS.RequestedPosition := 0;
   	            AXIS.RequestedVelocity := 0;
   	            AXIS.GeneralCommand := 16#80000061;
   	            IF NOT AXIS.AxisError.GeneralError  THEN
   	                State := 20;
   
   	            END_IF;
   
   
   	        20:
   	            AXIS.GeneralCommand := 16#0;
   	            State := 30;
   
   	        30:        //reset complete, reset to idle by setting execute false
   	            AXIS.GeneralCommand := 16#0;
   	            IF NOT Execute THEN
   	                State := 0;
   	            END_IF;
   
   	        80:     //Aborted by other command before completion
   	            IF NOT Execute THEN
   	                State := 0;
   	            END_IF;
   
   	        90:       //Error while disabling, reset to idle by setting execute false
   	            IF NOT Execute THEN
   	                State := 0;
   	            END_IF;
   
   	        ELSE
   	            State := 90;
   
   	    END_CASE;
   
   	//END_REGION
   
   	//REGION STATUS SIGNALS
   
   	    Done := State = 30;
   	    CommandAborted := State = 80;
   	    Busy := State <> 0 AND NOT Done AND NOT CommandAborted;
   
   	//END_REGION
   
END_ROUTINE
END_ADD_ON_INSTRUCTION

ADD_ON_INSTRUCTION MIS_Stop   (* revision 1.0 *)
VAR_IN_OUT
   AXIS : JVL_AXIS_MIS; {required}
END_VAR
VAR_OUTPUT
   CommandAborted : BOOL; {access Read Only, visible}
   Busy : BOOL; {access Read Only, visible}
   Done : BOOL; {access Read Only, visible}
   Error : BOOL; {access Read Only, visible}
END_VAR
VAR_INPUT
   Deceleration : REAL; {required}
   Execute : BOOL; {required}
END_VAR
VAR
   State : INT; {access None}
   ExecuteStart : BOOL; {access None}
   ActiveDeceleration : DINT; {access None}
   AOI_Type : DINT; {access None}
END_VAR

ROUTINE Logic   (* structured text *)
   	//REGION CAPTURE EDGES
   	    if Execute and not ExecuteStart then
   	    	ExecuteStart:=1;
   		elsif not Execute then
   			ExecuteStart:=0;
   		end_if;
   
   	//END_REGION
   
   	//REGION STATE CHANGES
   
   	    //Re-trigger sequence from start on rising edge
   
   	    //Command aborted
   	    IF AXIS.AOI_Type <> AOI_Type AND
   	        State <> 0 AND
   	        State <> 90 AND
   	        State <> 30 AND
   	        State <> 80
   	    THEN
   	        State := 80;
   	    END_IF;
   
   	    //Error if motor error while executing
   	    IF AXIS.AxisError.GeneralError AND
   	        State <> 0 AND
   	        State <> 90 AND
   	        State <> 30 AND
   	        State <> 80
   	    THEN
   	        State := 90;
   	    END_IF;
   
   	//END_REGION
   
   	//REGION STATE MACHINE
   
   	    CASE State OF
   
   	        0:        //Wait for rising edge on execute
   	            ActiveDeceleration := 0;
   
   	            IF ExecuteStart THEN
   					AOI_Type:= 6;
   					AXIS.AOI_Type:= 6;
   	                AXIS.RequestedMode:= 1;
   	                ActiveDeceleration :=  Deceleration;//
   	                //set Acceleration always >=1
   	                IF ActiveDeceleration < 1 THEN
   	                    ActiveDeceleration := 1;
   	                END_IF;
   	                State := 10;
   	            END_IF;
   
   	        10:        //Trigger stop
   	            IF AXIS.ActualMode = 1 THEN
   	                AXIS.RequestedDeceleration := ActiveDeceleration;
   	                AXIS.RequestedVelocity := 0;
   	                State := 20;
   
   	            ELSE            //Go to Idle if other command has changed the operating state
   	                State := 0;
   	            END_IF;
   
   	        20:    //Check stop is complete
   	            IF AXIS.RequestedMode = 1 AND
   	                AXIS.RequestedVelocity = 0 THEN
   
   	                //If no motion then stop is complete
   	                IF ABS(AXIS.ActualVelocity) <= 1.0 AND
   	                    NOT AXIS.AxisStatus.Accelerating and
   	                    //NOT AXIS.AxisStatus.AtVelocity and
   	                    NOT AXIS.AxisStatus.Decelerating THEN
   	                    State := 30;
   	                END_IF;
   
   	            ELSE            //Go to Idle if other command has changed the operating state
   	                State := 0;
   	            END_IF;
   
   	        30:        //Disable complete, reset to idle by setting execute false
   	            IF NOT Execute THEN
   	                State := 0;
   					ExecuteStart:=0;
   
   	            END_IF;
   
   	        80:     //Aborted by other command before completion
   	            IF NOT Execute THEN
   	                State := 0;
   					ExecuteStart:=0;
   	            END_IF;
   
   	        90:       //Error while disabling, reset to idle by setting execute false
   	            IF NOT Execute THEN
   	                State := 0;
   					ExecuteStart:=0;
   	            END_IF;
   
   	        ELSE
   	            State := 90;
   
   	    END_CASE;
   
   	//END_REGION
   
   	//REGION STATUS SIGNALS
   
   	    Done := State = 30;
   	    CommandAborted := State = 80;
   	    Error := State = 90;
   	    Busy := State <> 0 AND NOT Done AND NOT Error AND NOT CommandAborted;
   
   	//END_REGION
END_ROUTINE
END_ADD_ON_INSTRUCTION
